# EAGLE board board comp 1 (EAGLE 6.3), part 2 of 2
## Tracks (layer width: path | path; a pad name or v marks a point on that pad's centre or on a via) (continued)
BLINKER_R_FRONT_-  (via drill 0.61) (continued)
  Top 0.254: BLINKER-R1.4 258.95,42.42 | 258.95,42.42 BLINKER-R1.2 | v252.35,28.07 255.65,31.37 255.65,42.42 258.95,42.42
  Bottom 0.254: SV4.15 250.19,12.45 250.19,25.02 252.35,27.18 v252.35,28.07
  pour Top: 255.14,38.99 267.84,38.99 267.84,61.85 255.14,61.85
BRAKE  (via drill 0.61)
  Top 0.254: BRAKE-L1.1 230,41.02 231.39,42.42 237.36,42.42 238.76,41.02 BRAKE-C1.1 238.89,40.89 238.89,35.81 240.41,34.29 243.84,34.29 | 243.84,34.29 243.84,37.08 247.65,40.89 BRAKE-R1.1 | 244.35,27.18 246.13,27.18 247.52,25.78 R9.2 247.52,25.91 247.78,25.91 248.54,26.67 261.87,26.67 262.76,25.78 R16.2 | 244.35,27.18 222.12,27.18 | 222.12,27.18 218.44,27.18 217.04,25.78 R1.2 | v223.39,25.65 224.66,25.65 R3.2 | 222.12,27.18 v222.12,26.92 | 243.84,34.29 244.86,34.29 245.36,33.78 v245.36,29.72 | 244.35,27.18 v244.35,26.8
  Bottom 0.254: v222.12,26.92 v223.39,25.65 | v245.36,29.72 244.35,28.7 v244.35,26.8
BRAKE_C_-  (via drill 0.61)
  Top 0.254: v244.47,33.4 244.47,29.59 244.22,29.34 242.57,29.34 241.17,30.73 BRAKE-C2.2 | v242.95,35.18 241.17,36.96 BRAKE-C2.4 BRAKE-C1.2 BRAKE-C1.4 | SV4.7 240.03,12.45 242.19,12.45 v242.44,12.7
  Bottom 0.254: v242.95,35.18 242.95,34.92 v244.47,33.4 244.35,33.4 242.7,31.75 242.7,26.42 242.82,26.29 242.82,23.11 242.57,22.86 242.57,12.83 v242.44,12.7
  pour Top: 244.98,2.16 244.98,61.85 237.36,61.85 237.36,2.16
BRAKE_L_-  (via drill 0.61)
  Top 0.254: 232.28,39.5 BRAKE-L2.4 232.28,32.26 | 232.28,39.5 BRAKE-L1.2 | 232.28,32.26 BRAKE-L2.2 | v237.11,29.97 237.11,32.26 232.28,32.26 | 232.28,39.5 228.98,39.5 228.98,43.81 232.28,47.12 BRAKE-L1.4
  Bottom 0.254: SV4.9 239.78,12.45 239.78,27.3 v237.11,29.97
  pour Top: 236.09,2.16 236.09,61.85 228.47,61.85 228.47,2.16
BRAKE_R_-  (via drill 0.61)
  Top 0.254: SV4.5 234.7,12.45 234.7,15.49 236.35,15.49 242.44,21.59 v246,21.59 | v249.81,28.07 249.81,30.73 250.06,30.73 BRAKE-R2.2 BRAKE-R2.4 BRAKE-R1.2 BRAKE-R1.4
  Bottom 0.254: v246,21.59 249.81,25.4 v249.81,28.07
  pour Top: 253.87,2.16 253.87,61.85 246.25,61.85 246.25,2.16
BRAKE_REGEN  (via drill 0.61)
  Top 0.254: R2.2 220.85,25.78 221.11,26.04 222.5,26.04 223.01,26.54 227.71,26.54 228.47,25.78 R4.2 228.47,25.91 228.85,26.29 v229.62,26.29 | 231.58,29.15 231.65,29.08 237.49,29.08 238.76,30.35 238.76,30.73 BRAKE-C2.1 238.76,30.23 240.16,28.83 247.65,28.83 | 231.58,29.15 230,30.73 BRAKE-L2.1 | 231.58,29.15 v231.01,28.57 | v245.62,26.29 243.71,24.38 R8.1 | 247.65,28.83 247.65,30.73 BRAKE-R2.1 | 247.65,28.83 v247.65,28.32 248.79,27.18 265.18,27.18 266.57,25.78 R17.2
  Bottom 0.254: v229.62,26.29 231.01,27.69 v231.01,28.57 | v247.65,28.32 v245.62,26.29
CONTACTOR_IN
  Bottom 2.54: CONTACTOR.2 52.45,82.96 K3.S@
CONTACTOR_OUT
  Bottom 2.54: K3.P@ 48.64,87.63 56.26,87.63 56.26,64.14 CONTACTOR.1
CURRENT
  Top 0.254: R84.2 75.31,59.69 SV3.7
D5V+  (via drill 0.61)
  Top 0.254: L5.2 214.12,88.27 214.12,92.08 C53.2 213.64,92.18 C52.2 213.72,95.99 213.72,97.28 213.87,97.28 v218.36,101.78 | v233.45,117.47 233.83,117.09 234.14,117.09 235.03,116.2 R51.2 234.95,116.1 234.95,112.5 C51.2 235.28,112.39 235.28,107.95 U$2.P$27_ | v222.22,112.22 229.11,119.1 v231.88,119.1
  Bottom 0.254: R52.2 233.45,116.31 v233.45,117.47 233.38,117.58 233.38,117.6 v231.88,119.1 | v218.36,101.78 220.96,104.37 220.96,109.65 222.22,110.92 v222.22,112.22
DC+
  Top 0.254: S1.2 194.82,110.13 194.69,110.13 192.56,112.27 192.56,116.2 POWER.1
DGND0  (via drill 0.61)
  Top 0.254: JP11.18 219.15,78.11 220.8,79.76 227.25,79.76 228.91,78.11 JP11.10 229.31,78.11 230.96,79.76 232.99,79.76 | JP11.4 236.53,78.11 234.87,79.76 232.99,79.76 | U$2.P$28_ 235.81,107.95 235.81,108.51 236.45,109.14 C51.1 236.45,112.5 236.45,114.3 235.94,114.81 235.94,119.15 233.12,119.15 231.44,117.47 229.31,117.47 228.22,116.38 227.99,116.38 JP13.6 227.89,116.36 227.89,113.84 JP13.4 227.89,113.72 227.89,111.3 JP13.2 227.74,111.3 223.8,111.3 v222.17,109.68 | C52.1 C53.1 216.74,92.69 221.21,92.69 221.28,92.76 221.39,92.84 | 228.27,94.94 228.27,94.89 228.45,94.89 228.47,94.87 IC10.3 | 228.27,94.94 R53.1 228.27,98.53 228.27,98.7 228.93,99.36 231.19,99.36 231.19,96.06 231.01,95.89 IC10.1 | 228.27,94.94 227.2,94.94 IC10.4 227.1,94.61 223.44,94.61 | 221.39,92.84 222.71,91.52 228.57,91.52 229.39,90.7 229.74,90.7 IC10.7 229.74,88.88 230.63,87.99 231.67,87.99 232.08,88.39 234.77,88.39 234.77,87.2 234.29,86.72 233.66,86.72 233.66,83.08 232.99,82.42 232.99,79.76 | 221.39,92.84 221.39,93.55 222.45,94.61 223.44,94.61 | 223.44,94.61 v223.44,98.65
  Bottom 0.254: v222.17,109.68 222.22,109.63 222.22,99.87 v223.44,98.65
DIR
  Top 0.254: IO.2 160.87,128.78 164.68,124.97 R26.2
DM
  Top 0.254: IC5.7 195.59,9.08 CONN1.D-
DP
  Top 0.254: IC5.8 196.09,12.06 196.34,11.81 CONN1.D+
EECLK  (via drill 0.38)
  Top 0.254: IC5.62 193.97,33.7 v195.2,34.92
  Top 0.305: v190.37,53.21 190.5,53.09 IC7.2 194.06,53.09 194.69,52.45 v200.79,52.45 201.04,52.7 R32.1
  Bottom 0.254: v195.2,34.92 197.49,34.92 200.79,38.23 v200.79,52.45
  Bottom 0.305: JP3.21 189.99,53.59 v190.37,53.21
EECS  (via drill 0.38)
  Top 0.254: IC5.63 194.74,33.2 v195.2,33.66
  Top 0.305: v190.37,51.69 190.5,51.82 IC7.1 193.8,51.82 194.18,51.44 203.07,51.44 v203.45,51.82 203.58,51.94 R34.1
  Bottom 0.254: v195.2,33.66 197.23,33.66 203.33,40.01 203.33,51.69 v203.45,51.82
  Bottom 0.305: JP3.20 189.74,51.05 v190.37,51.69
EEDATA  (via drill 0.38)
  Top 0.254: IC5.61 192.95,34.2 195.2,36.45 v195.71,36.45
  Top 0.305: R31.2 194.5,53.91 194.06,54.36 IC7.3 190.75,54.36 v190.37,54.74
  Bottom 0.254: v195.71,36.45 197.49,36.45 199.52,38.48 199.52,50.16 194.94,54.74 v190.37,54.74
  Bottom 0.305: JP3.22 188.98,56.13 v190.37,54.74
GND  (via drill 0.61)
  Top 0.254: BRAKE-L1.3 234.7,40.89 v236.6,38.99 238.38,37.21 238.38,32.26 242.06,32.26 243.46,30.86 BRAKE-C2.3 | 232.28,24.38 v234.19,24.38 236.09,24.38 R6.1 | 220.85,24.38 217.04,24.38 R1.1 | 228.47,24.38 224.66,24.38 | 224.66,24.38 220.85,24.38 | 220.85,24.38 R2.1 | 224.66,24.38 R3.1 | 228.47,24.38 232.28,24.38 | 232.28,24.38 R5.1 | 228.47,24.38 R4.1 | BLINKER-R1.3 261.24,40.89 v261.24,35.18 261.24,30.86 BLINKER-R2.3 | BRAKE-R1.3 252.35,40.89 v252.35,35.18 252.35,30.86 BRAKE-R2.3 | BLINKER-L1.3 225.68,40.89 v225.68,35.18 225.68,30.86 BLINKER-L2.3 | 258.95,24.38 v257.05,24.38 255.14,24.38 R14.1 | 262.76,24.38 266.57,24.38 R17.1 | 262.76,24.38 258.95,24.38 | 258.95,24.38 R15.1 | 262.76,24.38 R16.1 | v244.86,40.89 243.59,40.89 BRAKE-C1.3 | v235.97,30.73 234.7,30.73 BRAKE-L2.3
  pour Bottom: 267.84,61.85 215.77,61.85 215.77,2.16 267.84,2.16
GND0  (via drill 0.61)
  Top 0.254: v215.14,108.2 R57.2 215.24,109.78 215.62,110.16 218.97,110.16 228.75,119.94 242.72,119.94 245.72,116.94 245.72,113.36 | v211.73,91.47 205.66,85.39 202.95,85.39 201.35,87 R56.2 | 251.71,85.24 259.66,85.24 X3.4 | 251.71,85.24 X3.5 | 251.71,85.24 251.71,78.23 252.68,77.27 254.97,77.27 259.66,72.57 X3.3 | 236.53,102.97 236.78,102.97 U$2.P$11_ | 236.53,102.97 U$2.P$12_ 236.27,102.84 236.27,98.42 C46.1 235.23,98.32 C47.1 235.33,94.54 237.06,92.81 243.56,92.81 243.56,88.67 v244.93,87.3 | 236.8,106.78 236.8,105.74 236.53,105.46 236.53,102.97 | 236.8,106.78 236.8,107.92 U$2.P$30_ | v236.91,106.78 236.8,106.78 | v248.56,112.95 248.56,113.36 245.72,113.36 | 245.72,113.36 240.72,113.36 v238.46,111.1
  Bottom 0.254: v215.14,108.2 213.72,106.78 213.72,95.99 C55.1 C54.1 213.51,92.02 212.95,91.47 v211.73,91.47 | R56.2 200.63,87 200.63,87.12 193.24,94.51 192.38,94.51 192.38,94.54 C57.2 192.28,95.35 192.38,95.45 192.38,97.26 C56.2 195.99,101.04 195.99,102.26 196.65,102.92 196.65,113.26 197.08,113.69 197.08,115.93 POWER.2 | 248.65,112.86 248.84,113.06 253.62,113.06 253.62,113.87 253.67,113.92 253.67,115.09 U$11.4 | 248.65,112.86 248.08,112.29 248.08,112.14 246.89,112.14 C45.1 | C48.1 235.41,109.63 C49.1 235.56,109.63 C50.1 | v236.91,106.78 237.39,107.26 237.39,109.53 C50.1 | v238.46,111.1 238.07,110.72 238.07,109.73 C50.1 | v248.56,112.95 248.65,112.86 | v244.93,87.3 246.96,85.27 X3.5
GND1
  pour Top: 1.65,1.27 99.44,1.27 99.44,50.8 1.65,50.8
GND4
  Top 0.254: U$3.2 216.1,116.36 216.1,112.55 215.14,112.55 R57.1
GND5  (via drill 0.38)
  Top 0.254: ADC_CAP3.2 139.22,46.74 139.79,46.16 | 139.79,46.16 143.76,42.19 ADC3.9 | 7805CAP1.2 108.71,56.26 108.71,52.55 7805CAP2.2 108.69,52.45 106.96,50.72 ADC_CAP1.2 107.06,46.15 119.23,46.15 121.58,43.8 | 126.99,49.14 127.99,50.14 129.01,50.14 | 126.99,49.14 124.08,46.23 ADC_CAP2.2 123.95,46.18 121.58,43.8 | 129.01,50.14 129.79,50.93 6103CAP2.2 129.87,51.03 130.18,51.33 130.18,54.63 3V.3 129.82,55.17 6103CAP1.2 129.92,58.62 131.29,59.99 142.26,59.99 317CAP2.2 142.37,60.07 145.54,60.07 146.43,59.18 317CAP1.2 146.48,59.05 149.22,56.31 R22.2 149.33,54.86 160.07,54.86 162.13,52.81 162.13,52.25 U$1.4 162.18,46.18 160.11,44.11 | 121.58,43.8 120.98,43.2 117.55,43.2 115.95,41.6 115.82,41.6 ADC1.9 | v130.71,42.52 129.79,41.6 ADC2.9 | 130.71,46.86 130.71,48.41 129.08,50.04 129.01,50.14 | 130.71,46.86 v130.71,46.18 | 130.71,46.86 v135.18,46.86 | v139.65,46.02 139.79,46.16 | 126.99,49.14 121.64,54.48 5V.3 | ADC_CAP4.2 154.15,46.23 157.73,42.65 ADC4.9 157.84,41.83 160.11,44.11 | 169.48,34.73 SV2.2 SV2.3 | 169.48,34.73 166.32,31.57 166.32,24.89 R23.2 166.24,24.79 166.24,15.34 160.27,9.37 SV1.33 | 169.48,34.73 160.11,44.11
  Bottom 0.254: v130.71,46.18 v130.71,42.52 | v139.65,46.02 136.02,46.02 v135.18,46.86
  pour Bottom: 103.12,40.77 103.12,70.61 176.78,70.61 176.78,1.4 165.99,1.4 165.99,40.77
  pour Top: 103.12,40.77 103.12,70.61 176.78,70.61 176.78,1.4 165.99,1.4 165.99,40.77
GND6
  Top 0.254: 169.13,118.62 169.13,119.89 164.05,119.89 162.78,118.62 T1.2 | 169.13,118.62 167.86,117.35 167.86,95.76 165.32,93.22 POWER1.1 | 169.13,118.62 T2.2
  Bottom 2.794: POWER1.1 156.43,92.58 156.43,95.76 137.05,95.76 K2.P2
GND7  (via drill 0.38)
  Top 0.254: IC5.15 199.59,32.64 v199.64,32.64 198.75,32.64 198.59,32.48 IC5.13 | IC5.11 197.59,32.02 197.49,32.13 194.94,32.13 194.59,31.78 IC5.5 | IC5.1 192.59,31.81 192.66,31.88 194.18,31.88 | IC5.47 193.09,43.13 192.91,43.31 v192.28,43.31 | IC5.51 196,39.2 196.22,38.99 196.22,38.1 v196.09,37.97 | IC5.35 199.09,40.68 199.26,40.51 200.28,40.51 200.91,41.15 v202.06,41.15 | IC5.25 208.66,36.7 210.19,35.18 | 197.1,30.86 197.1,31.88 | 198.59,30.9 198.59,29.7 199.35,28.94
  other vias: 204.72,15.88 207.77,15.88 209.04,11.56 197.99,12.57 198.88,8.51 207.77,30.1 203.96,19.68 190.75,29.34 188.72,23.5 205.23,22.73 190.25,17.91 202.18,43.81 202.18,49.66 191.9,6.1 189.48,10.41 198.75,22.99 199.9,28.07 192.02,11.18 194.18,4.32 197.99,4.06 196.22,1.78 201.55,12.19 188.85,6.1 202.31,57.15 207.65,57.15 206.63,41.91 208.41,42.16 202.31,31.5 185.29,47.24 182.75,54.86 185.04,55.12
  pour Bottom (isolate 0.305): 213.49,0.89 213.49,58.04 179.2,58.04 179.2,0.89
  pour Top (isolate 0.305): 213.49,0.89 213.49,58.04 179.2,58.04 179.2,0.89
GND8  (via drill 0.6)
  other vias: 65.15,113.03 43.56,100.33 66.42,119.38 62.61,77.47
  pour Top: 1.65,54.61 99.44,54.61 99.44,139.7 1.65,139.7
  pour Bottom: 1.65,54.61 99.44,54.61 99.44,139.7 1.65,139.7
IN1  (via drill 0.38)
  Top 0.254: 110.74,20.7 110.74,17.27 SV1.1 | 110.74,20.7 LMC6484_1.3 | v119.63,22.17 120.37,22.91 124.08,22.91 U$6.1 | 110.74,20.7 v118.16,20.7
  Bottom 0.254: v118.16,20.7 v119.63,22.17
IN2
  Top 0.254: LMC6484_1.5 113.28,22.58 114.43,21.44 119.63,21.44 | 119.63,21.44 124.46,21.44 125.35,22.33 U$6.2 | 119.63,21.44 SV1.2
IN3  (via drill 0.38)
  Top 0.254: SV1.3 123.27,9.47 123.27,11.02 126.62,14.38 U$6.3 126.57,23.04 126.57,23.6 125.53,24.64 v124.38,24.64 | LMC6484_1.10 113.28,27.76 114.55,26.49 v122.53,26.49
  Bottom 0.254: v124.38,24.64 v122.53,26.49
IN4  (via drill 0.38)
  Top 0.254: U$6.4 127.89,16.69 v127.36,16.15 | v124.51,13.31 124.51,13.26 SV1.4 | LMC6484_1.12 110.74,27.08 v112.93,24.89
  Bottom 0.254: v127.36,16.15 v124.51,13.31 v112.93,24.89
IN5  (via drill 0.38)
  Top 0.254: U$6.5 129.16,16.41 v128.35,15.6 | ADC1.5 112.01,35.79 v119.84,27.96
  Bottom 0.254: SV1.5 125.81,9.47 127.36,9.47 128.35,10.46 v128.35,15.6 128.27,15.7 128.27,21.79 122.1,27.96 v119.84,27.96
IN6  (via drill 0.38)
  Top 0.254: SV1.6 130.43,16.64 U$6.6 130.38,23.04 130.38,23.6 v129.34,24.64 | ADC1.6 113.28,35.79 v120.12,28.96
  Bottom 0.254: v120.12,28.96 125.02,28.96 v129.34,24.64
IN7  (via drill 0.38)
  Top 0.254: SV1.7 128.35,9.47 128.35,11.02 131.93,14.61 131.93,21.01 131.7,21.23 U$6.7 131.65,23.04 131.65,23.6 v130.43,24.82 | ADC1.7 114.55,35.79 v120.4,29.95
  Bottom 0.254: v120.4,29.95 125.3,29.95 v130.43,24.82
IN8  (via drill 0.38)
  Top 0.254: ADC1.8 115.82,35.56 v116.61,34.77 | v132.97,25.91 U$6.9 | v131.19,20.7 131.19,14.86 SV1.8
  Bottom 0.254: v116.61,34.77 116.61,24.77 116.18,24.33 114.53,24.33 113.23,25.63 112.62,25.63 112.19,25.2 112.19,24.59 124.77,12.01 126.16,12.01 SV1.8 | v132.97,25.91 132.97,22.48 v131.19,20.7
IN9  (via drill 0.38)
  Top 0.254: v131.7,30.61 U$6.10 | v121.54,38 121.54,37.03 ADC2.1
  Bottom 0.254: v131.7,30.61 131.7,30.89 128.08,34.51 | 128.08,34.51 124.59,38 v121.54,38 | SV1.9 130.78,8.38 132.23,9.83 135.33,9.83 136.32,10.82 136.32,15.14 142.09,20.9 142.09,23.6 131.09,34.59 128.17,34.59 128.08,34.51
IN10  (via drill 0.38)
  Top 0.254: v130.43,26.42 U$6.11 | v122.17,34.65 ADC2.2
  Bottom 0.254: SV1.10 129.79,23.11 131.17,24.49 131.17,25.12 130.43,25.86 v130.43,26.42 130.33,26.49 v122.17,34.65
IN11
  Top 0.254: ADC2.3 123.44,37.01 124.92,38.48 130.53,38.48 131.19,37.82 131.19,32.05 | 131.19,32.05 131.19,31.14 129.16,29.11 U$6.12 | SV1.11 132.33,9.37 133.66,10.69 133.66,25.65 133.71,25.7 133.71,29.64 131.29,32.05 131.19,32.05
IN12  (via drill 0.38)
  Top 0.254: 127.89,29.84 127.89,30.91 130.53,33.55 130.53,37.54 130.25,37.82 125.53,37.82 124.71,37.01 ADC2.4 | 127.89,29.84 U$6.13 | v128.04,29.84 127.89,29.84
  Bottom 0.254: SV1.12 132.33,18.52 130.45,20.4 130.45,22.84 131.83,24.21 131.83,26.06 v128.04,29.84
IN13  (via drill 0.38)
  Top 0.254: ADC2.5 125.98,34.52 126.62,33.88 U$6.14 126.57,28.02 126.57,27.46 125.81,26.7 123.62,26.7 123.09,27.23 v121.08,27.23 | SV1.13 133.88,8.38 132.79,7.29 121.72,7.29 121.08,7.92 v121.08,20.7
  Bottom 0.254: v121.08,27.23 v121.08,20.7
IN14  (via drill 0.38)
  Top 0.254: v125.35,33.15 U$6.15 | v126.87,34.67 126.87,35.99 127.25,36.37 ADC2.6
  Bottom 0.254: v126.87,34.67 126.21,34.01 | 126.21,34.01 v125.35,33.15 | SV1.14 134.87,22.12 135.13,22.38 135.13,25.09 126.21,34.01
IN15  (via drill 0.38)
  Top 0.254: SV1.15 136.32,9.47 136.32,11.38 138.05,13.11 U$7.1 138,23.04 137.13,23.9 v137.13,24.13 | v128.52,32.74 ADC2.7
  Bottom 0.254: v137.13,24.13 v128.52,32.74
IN16  (via drill 0.38)
  Top 0.254: SV1.16 139.32,12.83 U$7.2 139.27,23.04 138.96,23.34 v138.96,24.64 | v129.79,33.86 ADC2.8
  Bottom 0.254: v129.79,33.86 129.79,33.81 v138.96,24.64
IN17  (via drill 0.38)
  Top 0.254: SV1.17 138.86,9.47 138.86,11.38 140.59,13.11 U$7.3 140.54,23.04 140.03,23.55 v140.03,24.61 | v134.87,29.77 ADC3.1
  Bottom 0.254: v140.03,24.61 v134.87,29.77
IN18  (via drill 0.38)
  Top 0.254: 141.86,21.21 141.86,12.83 SV1.18 | 141.86,21.21 U$7.4 | v136.14,26.42 ADC3.2 | 141.86,21.21 v141.35,21.21
  Bottom 0.254: v141.35,21.21 v136.14,26.42
IN19  (via drill 0.38)
  Top 0.254: SV1.19 141.4,9.47 141.4,11.38 143.13,13.11 U$7.5 143.08,23.04 142.54,23.57 v142.54,24.61 | v137.41,29.74 ADC3.3
  Bottom 0.254: v142.54,24.61 v137.41,29.74
IN20  (via drill 0.38)
  Top 0.254: SV1.20 144.4,12.83 U$7.6 144.35,23.04 144.35,23.6 143.56,24.38 v143.56,24.64 | v138.68,32.05 ADC3.4
  Bottom 0.254: v138.68,32.05 139.37,31.37 139.37,30.4 139.12,30.15 139.12,29.08 v143.56,24.64
IN21  (via drill 0.38)
  Top 0.254: SV1.21 143.94,9.47 143.94,11.38 145.67,13.11 U$7.7 145.62,23.04 145.62,23.62 v144.6,24.64 | ADC3.5 139.95,31.7 v140.08,31.57
  Bottom 0.254: v140.08,31.57 140.08,29.16 v144.6,24.64
IN22  (via drill 0.38)
  Top 0.254: U$7.9 146.94,29.79 v145.8,30.94 | v143.66,33.07 143.66,33.17 141.22,35.61 ADC3.6 | SV1.22 145.03,11.53 146.41,12.9 v146.41,17.68
  Bottom 0.254: v143.66,33.07 144.21,32.52 | 144.21,32.52 v145.8,30.94 | v146.41,17.68 146.41,24.79 141.76,29.44 141.76,30.07 144.21,32.52
IN23  (via drill 0.38)
  Top 0.254: U$7.10 145.67,30.02 145.06,30.63 145.06,31.24 145.49,31.67 146.1,31.67 147.6,30.18 147.6,29.11 148.03,28.68 148.64,28.68 | 148.64,28.68 149.07,29.11 149.07,31.37 144.42,36.02 144.42,37.62 144.22,37.82 143.31,37.82 142.49,37.01 ADC3.7 | v148.67,28.42 148.67,28.57 148.64,28.68
  Bottom 0.254: SV1.23 147.57,9.37 148.67,10.46 v148.67,28.42
IN24  (via drill 0.38)
  Top 0.254: 144.4,32.33 144.4,35.1 143.76,35.74 ADC3.8 | 144.4,32.33 U$7.11 | v148.34,29.41 148.34,30.38 146.38,32.33 144.4,32.33
  Bottom 0.254: SV1.24 147.57,28.65 v148.34,29.41
IN25  (via drill 0.38)
  Top 0.254: U$7.12 143.13,29.31 v143.66,29.84 | v148.9,34.67 148.9,36.32 148.84,36.37 ADC4.1
  Bottom 0.254: v143.66,29.84 145.75,29.84 148.9,32.99 148.9,34.01 | v148.9,34.67 148.9,34.01 | SV1.25 150.11,9.37 151.21,10.46 151.21,33.22 150.42,34.01 148.9,34.01
IN26  (via drill 0.38)
  Top 0.254: U$7.13 141.86,29.11 v142.49,29.74 | ADC4.2 v150.11,33.27
  Bottom 0.254: v142.49,29.74 142.72,29.74 143.36,29.11 145.95,29.11 147.81,30.98 | v150.11,33.27 147.81,30.98 | SV1.26 150.11,28.68 147.81,30.98
IN27  (via drill 0.38)
  Top 0.254: U$7.14 140.59,31.04 v142.67,33.12 | v150.85,34.67 150.85,35.84 151.38,36.37 ADC4.3 151.28,36.45 151.28,38.3 151.71,38.73 v154.31,38.73
  Bottom 0.254: v142.67,33.12 144.96,35.41 150.11,35.41 v150.85,34.67 | SV1.27 153.65,8.38 154.74,7.29 160.73,7.29 161.37,7.92 161.37,31.67 v154.31,38.73
IN28  (via drill 0.38)
  Top 0.254: U$7.15 139.32,30.38 v138.63,31.06 | v152.76,34.67 152.76,36.27 152.65,36.37 ADC4.4
  Bottom 0.254: v138.63,31.06 137.95,31.75 137.95,32.36 143.26,37.67 150.65,37.67 151.71,38.73 152.32,38.73 152.76,38.3 v152.76,34.67 152.76,24.51 152.65,24.41 SV1.28
IN29  (via drill 0.38)
  Top 0.254: U$8.1 152.02,14.15 v154.1,12.06 | v153.92,34.29 ADC4.5
  Bottom 0.254: SV1.29 154.1,9.47 v154.1,12.06 154.03,12.17 153.92,12.27 v153.92,34.29
IN30  (via drill 0.38)
  Top 0.254: SV1.30 155.19,12.01 153.29,13.92 U$8.2 153.24,23.04 153.24,23.6 v152.02,24.82 | ADC4.6 155.19,37.01 154.2,38 v152.02,38
  Bottom 0.254: v152.02,24.82 v152.02,38
IN31  (via drill 0.38)
  Top 0.254: ADC4.7 156.46,35.79 153.92,33.25 153.92,26.87 154.56,26.24 U$8.3 154.61,22.81 154.61,22.28 v156.29,20.6
  Bottom 0.254: SV1.31 157.73,9.37 156.29,10.82 v156.29,20.6
IN32  (via drill 0.38)
  Top 0.254: U$8.5 155.83,33.88 157.73,35.79 ADC4.8 157.78,36.5 158.37,37.08 v158.37,38 | v158.37,43.41 U$1.1
  Bottom 0.254: v158.37,38 v158.37,43.41
MOTOR+
  Top 2.794: OUTPUT.2 142.46,133.86 D2.C
MOTOR+_PRE
  Bottom 2.794: K1.O2 132.06,83.19 132.06,86.98 142.05,86.98 K1.S1 152.62,90.68 152.62,88.14 171.67,88.14 171.67,104.65 157.7,104.65 D2.A
MOTOR-
  Top 2.794: OUTPUT.1 118.33,133.86 D1.C
MOTOR-_PRE
  Top 2.794: D1.A 132.07,117.35 K1.O1
  Bottom 2.794: K1.O1 128.49,90.68 128.49,79.25 142.05,79.25 K1.S2
N$1
  Top 0.254: SV4.2 231.01,17.53 236.98,23.5 236.98,24.13 239.27,26.42 240.54,26.42 241.05,25.91 243.59,25.91 243.71,25.78 R8.2
N$2  (via drill 0.61)
  Top 0.254: v232.16,15.11 232.16,17.91 239.9,25.65 R7.2
  Bottom 0.254: v232.16,15.11 233.55,13.72 SV4.4
N$3  (via drill 0.61)
  Top 0.254: v241.94,23.5 246.76,23.5 247.52,24.26 R9.1 | v240.66,22.23 233.17,14.73 233.04,14.73 232.16,13.84 232.16,11.05 SV4.1
  Bottom 0.254: v240.66,22.23 v241.94,23.5
N$4  (via drill 0.61)
  Top 0.254: v249.05,23.37 250.44,23.37 251.33,24.26 R10.1 | v247.27,21.59 240.54,14.86 v236.98,14.86
  Bottom 0.254: v247.27,21.59 v249.05,23.37 | v236.98,14.86 235.33,14.86 235.33,14.48 234.7,13.84 234.7,12.32 233.55,11.18 SV4.3
N$5
  Top 0.254: R11.2 4.19,29.97 | 4.19,29.97 R12.1 | 4.19,29.97 6.86,29.97 IC2.1
N$6
  Top 0.254: R13.2 70.23,38.86 | 70.23,38.86 R18.1 | 70.23,38.86 72.9,38.86 IC1.1
N$7
  Top 0.254: R20.1 96.9,30.99 | 96.9,30.99 R19.2 | 96.9,30.99 94.23,30.99 IC3.1
N$8
  Top 0.254: R21.2 138.43,53.39 IC4.1 141.55,50.44 144.15,53.03 149.22,53.03 R22.1
N$9
  Top 2.794: K1.P2 137.12,83.19 137.12,79.01 146.27,79.01 146.27,107.19 K2.S1
N$10
  Top 2.794: K1.P1 137.38,90.68 137.38,95.76 142.05,95.76 K2.S2
N$11
  Top 0.254: R24.1 151.35,112.27 150.84,112.78 133.82,112.78 133.82,89.53 127.47,83.19 K1.1
N$12  (via drill 0.61)
  Top 0.254: v168.75,102.49 168.75,111.38 169.63,112.27 R25.1
  Bottom 0.254: v168.75,102.49 168.36,102.11 119.47,102.11 K2.1
N$13
  Top 0.254: K1.2 127.22,100.84 127.22,136.4 143.73,136.4 164.05,116.08 T1.1
N$14  (via drill 0.61)
  Top 0.254: v169.13,116.08 170.4,116.08 T2.1
  Bottom 0.254: v169.13,116.08 165.32,119.89 129.76,119.89 K2.2
N$15
  Top 0.254: T2.3 171.28,118.36 169.76,119.89 R27.1
N$16  (via drill 0.61)
  Top 0.254: T1.3 167.47,118.36 v167.47,119 | v167.47,120.9 163.41,124.97 R26.1
  Bottom 0.254: v167.47,120.9 v167.47,119
N$17
  Top 0.254: IC5.6 195.09,17.29 193.93,16.13 R29.2
N$18
  Top 0.254: IC5.2 193.09,28.88 191.64,27.43 191.64,26.29 X1.1
  Top 0.305: C11.1 188.34,26.8 188.59,26.54 191.39,26.54 191.64,26.29
N$19
  Top 0.254: IC5.3 193.59,21.25 193.04,20.7 X1.2
  Top 0.305: C12.1 188.41,19.75 188.59,19.94 188.59,20.19 191.13,20.19 X1.2
N$20
  Top 0.406: PWR.C R28.2
N$21
  Top 0.305: R35.2 RX.C
N$22
  Top 0.305: R36.2 TX.C
N$23
  Top 0.254: U$2.P$1_ 238.53,107.21 243,111.68 250.39,111.68 C41.1 250.8,112.06 252.04,112.06 252.37,112.39 R40.2
N$24
  Top 0.254: U$2.P$2_ 238.53,106.7 247.17,106.7 250.7,110.24 C41.2 250.8,110.16 252.07,110.16 252.37,109.86 R41.2
N$25
  Top 0.254: U$2.P$3_ 238.53,106.2 250.16,106.2 250.7,105.66 C42.1 250.8,105.59 251.23,105.16 253.19,105.16 254.08,106.05 R42.2
N$26  (via drill 0.61)
  Top 0.254: v237.36,105.11 237.95,105.69 238.51,105.69 U$2.P$4_ | v238.68,102.84 238.96,102.56 249.38,102.56 250.7,103.89 C42.2 250.67,103.68 251.74,102.62 253.19,102.62 254.08,103.5 R43.2
  Bottom 0.254: v237.36,105.11 238.68,103.78 v238.68,102.84
N$27  (via drill 0.61)
  Top 0.254: v244.98,105.21 238.53,105.21 U$2.P$5_ | v245.09,100.89 245.39,100.58 250.7,100.58 C43.1 250.8,100.66 252.07,100.66 252.37,100.97 R44.2
  Bottom 0.254: v244.98,105.21 245.09,105.11 v245.09,100.89
N$28  (via drill 0.61)
  Top 0.254: v249.4,104.24 244.75,104.24 244.3,104.7 238.53,104.7 U$2.P$6_ | v249.5,99.75 250.42,98.83 250.7,98.83 C43.2 250.8,98.75 252.04,98.75 252.37,98.42 R45.2
  Bottom 0.254: v249.4,104.24 249.66,103.99 249.66,99.9 v249.5,99.75
N$29  (via drill 0.61)
  Top 0.254: v248.51,103.4 244.93,103.4 244.09,104.24 242.29,104.24 242.26,104.22 238.53,104.22 U$2.P$7_ | v248.82,101.73 248.94,101.85 253.03,101.85 253.24,101.65 253.24,95.89 R46.2 252.27,95.83 251.03,95.83 250.7,95.5 C44.1
  Bottom 0.254: v248.51,103.4 248.82,103.1 v248.82,101.73
N$30  (via drill 0.61)
  Top 0.254: v242.65,103.4 242.37,103.68 238.53,103.68 U$2.P$8_ | v243.56,100.89 250.7,93.75 C44.2 250.8,93.67 252.04,93.67 252.37,93.34 R47.2
  Bottom 0.254: v242.65,103.4 243.56,102.49 v243.56,100.89
N$31  (via drill 0.61)
  Top 0.254: 251.66,116.94 251.66,118.75 JP7.1 | 251.66,116.94 251.66,114.81 254.08,112.39 R40.1 | 251.66,116.94 v249.81,116.94
  Bottom 0.254: R48.2 249.83,118.75 249.81,118.72 v249.81,116.94 249.81,116.36 249.86,116.31 249.86,115.11 U$11.1
N$32
  Bottom 0.254: R48.1 251.54,118.75 251.44,118.64 251.44,117.2 251.08,116.84 251.08,116.36 251.13,116.31 251.13,115.11 U$11.2
N$33  (via drill 0.61)
  Top 0.254: v252.5,116.94 252.55,116.99 260.38,116.99 JP7.3
  Bottom 0.254: v252.5,116.94 252.5,115.19 U$11.3
N$34  (via drill 0.61)
  Top 0.254: JP8.1 257.05,112.8 254.1,109.86 R41.1 254.03,109.96 v252.86,111.12
  Bottom 0.254: R49.2 251.1,104.78 251.08,104.8 251.08,106.66 251.16,106.73 251.16,107.92 U$11.7 251.18,108.05 251.23,108.1 251.23,109.5 v252.86,111.12
N$35
  Bottom 0.254: R49.1 252.81,104.78 252.71,104.88 252.71,106.17 252.5,106.38 252.5,106.66 252.43,106.73 252.43,107.92 U$11.6
N$36  (via drill 0.61)
  Top 0.254: v254.71,107.92 255.09,107.54 262,107.54 262.61,108.15 262.61,114.94 JP8.3
  Bottom 0.254: v254.71,107.92 253.69,107.92 U$11.5
N$37
  Top 0.254: JP14.2 259.97,106.93 253.29,106.93 R42.1
N$38
  Top 0.254: JP14.1 259.97,104.39 253.29,104.39 R43.1
N$39
  Top 0.254: JP15.4 R44.1
N$40
  Top 0.254: JP15.3 R45.1
N$41
  Top 0.254: JP15.2 R46.1
N$42
  Top 0.254: JP15.1 R47.1
N$43  (via drill 0.61)
  Top 0.254: 237.79,100.89 237.79,98.42 C46.2 | 237.79,100.89 U$2.P$9_ | 237.79,100.89 v240.41,100.89
  Bottom 0.254: JP9.2 239.27,114.94 239.27,114.45 240.41,113.31 v240.41,100.89
N$44  (via drill 0.61)
  Top 0.254: v244.86,112.52 242.37,112.52 237.79,107.95 U$2.P$32_ | v244.88,116.59 242.95,118.52 239.04,118.52 JP9.1
  Bottom 0.254: v244.86,112.52 244.88,112.55 v244.88,116.59
N$45
  Top 0.305: IC7.4 196.15,55.63 R31.1 196.66,55.56 197.23,54.99 197.23,54.23 197.49,53.98 198.25,53.98 R33.1
N$46
  Top 0.254: JP10.2 240.06,117.47 240.06,114.07 237.31,111.33 237.31,107.95 U$2.P$31_
N$47  (via drill 0.61)
  Top 0.254: 237.13,96.62 237.13,94.61 C47.2 | 237.13,96.62 237.13,100 237.29,100.15 U$2.P$10_ | v241.81,100.89 239.32,98.4 239.32,96.62 237.13,96.62
  Bottom 0.254: JP10.1 242.59,114.15 242.59,113.77 243.81,112.55 243.81,112.32 244.88,111.25 244.88,106.83 241.81,103.76 v241.81,100.89
N$48
  Top 0.254: IC5.4 194.09,19.09 191.13,16.13 C16.1
  Top 0.406: C16.1 191.46,15.05 191.13,15.37 189,15.37 | 188.7,15.37 C14.+ 189,15.37 | L2.1 186.91,14.95 187.32,15.37 188.7,15.37 | 189,15.37 188.7,15.37
N$49
  Top 0.254: IC5.9 196.59,23.37 197.87,22.1 C15.1 197.93,20.38 198.25,20.7
  Top 0.305: 198.25,20.7 199.79,20.7 C13.+ 200.05,20.93 200.28,20.7 201.76,20.7 L1.1
N$50  (via drill 0.61)
  Top 0.254: v234.72,105.11 234.11,105.72 U$2.P$21_ | v242.72,91.24 242.72,75.64 240.16,75.64 240.08,75.56 JP11.1
  Bottom 0.254: v234.72,105.11 244.88,94.94 244.88,93.12 244.37,92.61 242.54,92.61 242.54,91.42 v242.72,91.24
N$51  (via drill 0.61)
  Top 0.254: v231.93,106.86 232.56,106.22 233.55,106.22 U$2.P$22_
  Bottom 0.254: v231.93,106.86 231.65,106.58 R50.1
N$52
  Top 0.254: JP11.5 234.26,75.64 235.84,75.64 235.91,75.56 JP11.3
  Bottom 0.254: JP11.3 236.73,75.46 237.74,74.45 237.74,73.91 239.95,73.91 242.34,76.3 242.34,90.42 241.88,90.88 241.88,91.9 231.83,101.96 231.83,103.73 231.65,103.91 R50.2
N$53  (via drill 0.61)
  Top 0.254: JP11.9 229.18,75.64 230.76,75.64 230.84,75.56 JP11.7 | JP12.1 229.87,107.31 231.95,105.23 233.55,105.23 U$2.P$20_ | v232.03,89.23 232.03,99.9 v226.64,99.9
  Bottom 0.254: JP11.7 233.15,77.06 233.15,78.54 233.3,78.69 233.3,78.79 231.6,80.49 231.6,88.8 v232.03,89.23 | v226.64,99.9 225.43,101.12 225.43,105.49 227.25,107.31 JP12.1
N$54  (via drill 0.61)
  Top 0.254: v230.35,103.68 230.86,104.19 233.55,104.19 U$2.P$18_
  Bottom 0.254: v230.35,103.68 230.15,103.48 230.15,102.74 230.91,101.98 230.91,95.66 228.32,93.07 228.32,79.65 227.46,78.79 227.46,78.69 227.61,78.54 227.61,77.67 227.46,77.52 227.46,77.32 227.58,77.19 227.58,76.78 226.57,75.77 JP11.11
N$55  (via drill 0.61)
  Top 0.254: v231.9,113.56 231.9,113.03 233.68,111.25 234.29,111.25 234.29,107.95 U$2.P$25_ | v227.91,109.86 227.31,109.25 224.51,109.25 222.02,106.76 222.02,102.03 v221.39,102.03
  Bottom 0.254: v231.9,113.56 231.47,113.56 231.47,113.41 230.4,112.34 229.82,112.34 229.82,112.19 228.93,111.3 228.93,110.87 v227.91,109.86 | v221.39,102.03 221.77,101.65 221.77,99.67 222.22,99.21 222.22,84.33 224.89,81.66 224.89,78.72 225.07,78.54 225.07,77.67 224.92,77.52 224.92,77.32 225.04,77.19 225.04,76.78 224.03,75.77 JP11.13
N$56  (via drill 0.61)
  Top 0.254: v234.72,106.5 234.31,106.5 234.14,106.68 233.6,106.68 U$2.P$23_ | v234.26,100.71 234.26,100.15 233.66,99.54 v233.66,89.23 | v232.44,87.55 227.33,82.45 225.81,82.45 v223.95,80.59
  Bottom 0.254: v234.72,106.5 233.88,105.66 233.88,103.58 234.26,103.2 v234.26,100.71 | v233.66,89.23 232.44,88.01 v232.44,87.55 | v223.95,80.59 222.99,79.63 222.99,77.67 223.14,77.52 223.14,77.42 221.49,75.77 JP11.15
N$57  (via drill 0.61)
  Top 0.254: v229.82,106.17 231.27,104.72 233.55,104.72 U$2.P$19_
  Bottom 0.254: v229.82,106.17 228.42,104.78 JP12.2
N$58  (via drill 0.61)
  Top 0.254: v227.48,86.69 223.24,82.45 221.82,82.45 217.91,78.54 217.91,76.38 217.93,76.38 218.75,75.56 JP11.17
  Bottom 0.254: JP12.3 227.48,101.88 v227.48,86.69
N$59  (via drill 0.61)
  Top 0.254: v229.13,109.88 228.04,108.79 224.71,108.79 224.71,104.5 225.48,103.73 229.11,103.73 230.84,102.01 234.29,102.01 U$2.P$16_
  Bottom 0.254: v229.13,109.88 230.4,111.15 230.4,111.28 JP13.1
N$60  (via drill 0.61)
  Top 0.254: v233.43,102.84 233.55,102.84 233.55,103.68 U$2.P$17_ | v233.4,108.23 233.4,110.87 230.45,113.82 230.43,113.82 JP13.3 230.78,113.67 233.32,116.2 R51.1
  Bottom 0.254: v233.43,102.84 233.4,102.87 v233.4,108.23
N$61  (via drill 0.61)
  Top 0.254: U$2.P$24_ 233.55,107.21 233.38,107.39 232.82,107.39 229.36,110.85 229.36,116.36 230.4,116.36 JP13.5 230.53,116.41 231.04,116.41 232.94,118.31 234.11,118.31 v234.95,117.47
  Bottom 0.254: v234.95,117.47 234.95,116.28 235.03,116.2 R52.1
N$62
  Top 0.254: JP11.20 216.46,78.11 216.46,78.87 221.72,84.12 221.87,84.12 227.2,89.46 IC10.5
N$63  (via drill 0.61)
  Top 0.254: v222.07,83.29 226.31,87.53 227.84,87.53 227.84,88.82 228.47,89.46 IC10.6
  Bottom 0.254: v222.07,83.29 222.02,83.24 222.02,80.06 221.41,79.45 221.41,78.99 221.49,78.92 JP11.16
N$64  (via drill 0.61)
  Top 0.254: C57.1 194.72,87.1 196.52,87.1 196.62,87 R55.1 197.46,87.07 198.98,88.59 203.2,88.59 204.8,87 R54.1 | v215.14,89.28 216.15,88.27 L5.1
  Bottom 0.254: v215.14,89.28 215.14,89.26 L6.2 214.02,88.21 206.81,88.21 | 206.81,88.21 205.97,88.21 205.97,88.01 204.98,87.02 R54.1 | IC15.2 206.4,102.08 206.4,100.13 206.81,99.72 206.81,88.21
N$65
  Top 0.254: R55.2 197.46,97.26 200.33,97.26 200.43,97.16 R56.1
  Bottom 0.254: IC15.1 203.56,102.08 203.56,100.13 201.17,97.74 R56.1
N$66
  Top 0.254: C56.1 191.01,101.5 191.26,101.5 198.35,108.58 S1.1
  Bottom 0.254: IC15.3 208.08,102.95 208.08,103.76 203.35,108.48 198.63,108.48 S1.1
N$67
  pour Bottom: 221.49,121.28 221.49,83.19 188.47,83.19 188.47,121.28
N$68
  pour Top: 221.49,121.28 221.49,83.19 188.47,83.19 188.47,121.28
N$69
  pour Bottom: 263.4,92.08 263.4,67.94 243.08,67.94 243.08,92.08 245.62,92.08 245.62,120.02 255.78,120.02 255.78,92.08
  pour Bottom: 255.78,92.08 259.59,92.08 259.59,113.67 255.78,113.67
N$70
  pour Bottom: 244.35,120.02 244.35,93.34 241.81,93.34 241.81,83.19 222.76,83.19 222.76,120.02
N$71
  pour Bottom: 241.81,81.92 241.81,67.94 189.74,67.94 189.74,81.92
N$72
  pour Top: 241.81,90.81 241.81,67.94 189.74,67.94 189.74,81.92 234.19,81.92 234.19,90.81
N$73
  pour Top: 240.54,109.86 240.54,100.97 231.65,100.97 231.65,109.86
N$74
  Top 0.508: U$5.P$1 NEWBATT.P$2
  Bottom 0.508: OLDBATT.P$2 U$5.P$1
N$75
  Top 0.508: U$9.P$1 NEWBATT.P$1
  Bottom 0.508: OLDBATT.P$1 U$9.P$1
N$76
  pour Top: 186.56,124.71 186.56,138.94 196.22,138.94 196.22,124.71
N$77
  pour Bottom: 186.56,124.71 186.56,138.94 196.22,138.94 196.22,124.71
N$78
  Top 0.508: U$10.P$1 NEWBATT1.P$2
  Bottom 0.508: OLDBATT1.P$2 U$10.P$1
N$79
  Top 0.508: U$12.P$1 NEWBATT1.P$1
  Bottom 0.508: OLDBATT1.P$1 U$12.P$1
N$80
  pour Top: 198.63,124.71 198.63,138.94 208.28,138.94 208.28,124.71
N$81
  pour Bottom: 198.63,124.71 198.63,138.94 208.28,138.94 208.28,124.71
N$82
  Top 0.508: U$13.P$1 NEWBATT2.P$2
  Bottom 0.508: OLDBATT2.P$2 U$13.P$1
N$83
  Top 0.508: U$14.P$1 NEWBATT2.P$1
  Bottom 0.508: OLDBATT2.P$1 U$14.P$1
N$84
  pour Top: 210.57,124.71 210.57,138.94 220.22,138.94 220.22,124.71
N$85
  pour Bottom: 210.57,124.71 210.57,138.94 220.22,138.94 220.22,124.71
N$86
  Top 0.508: U$15.P$1 NEWBATT3.P$2
  Bottom 0.508: OLDBATT3.P$2 U$15.P$1
N$87
  Top 0.508: U$16.P$1 NEWBATT3.P$1
  Bottom 0.508: OLDBATT3.P$1 U$16.P$1
N$88
  pour Top: 222.38,124.71 222.38,138.94 232.03,138.94 232.03,124.71
N$89
  pour Bottom: 222.38,124.71 222.38,138.94 232.03,138.94 232.03,124.71
N$90
  Top 0.508: U$17.P$1 NEWBATT4.P$2
  Bottom 0.508: OLDBATT4.P$2 U$17.P$1
N$91
  Top 0.508: U$18.P$1 NEWBATT4.P$1
  Bottom 0.508: OLDBATT4.P$1 U$18.P$1
N$92
  pour Top: 234.19,124.71 234.19,138.94 243.84,138.94 243.84,124.71
N$93
  pour Bottom: 234.19,124.71 234.19,138.94 243.84,138.94 243.84,124.71
N$94
  Top 0.508: U$19.P$1 NEWBATT5.P$2
  Bottom 0.508: OLDBATT5.P$2 U$19.P$1
N$95
  Top 0.508: U$20.P$1 NEWBATT5.P$1
  Bottom 0.508: OLDBATT5.P$1 U$20.P$1
N$96
  pour Top: 245.75,124.71 245.75,138.94 255.4,138.94 255.4,124.71
N$97
  pour Bottom: 245.75,124.71 245.75,138.94 255.4,138.94 255.4,124.71
N$98
  Top 0.508: U$21.P$1 NEWBATT6.P$2
  Bottom 0.508: OLDBATT6.P$2 U$21.P$1
N$99
  Top 0.508: U$22.P$1 NEWBATT6.P$1
  Bottom 0.508: OLDBATT6.P$1 U$22.P$1
N$100
  pour Top: 257.3,124.71 257.3,138.94 266.95,138.94 266.95,124.71
N$101
  pour Bottom: 257.3,124.71 257.3,138.94 266.95,138.94 266.95,124.71
N$169  (via drill 0.38)
  Top 0.254: v62.36,94.89 61.44,93.98 IC12.7
  Bottom 0.254: v62.36,94.89 74.24,94.89 78.56,99.21 90.4,99.21 UNDER_WARN.2
N$170  (via drill 0.38)
  Top 0.254: IC12.5 60.12,91.44 58.9,90.22 58.9,86.31 59.97,85.24 62.81,85.24 68.3,90.73 68.3,107.95 v69.06,108.71
  Bottom 0.254: v69.06,108.71 75.36,108.71 87.3,120.65 UNDER_CRIT.2
N$171  (via drill 0.38)
  Top 0.254: IC12.11 54.94,90.17 54.28,90.83 54.28,92.05 54.94,92.71 IC12.9 56.31,92.76 57.53,92.76 v57.94,93.17
  Bottom 0.254: TEMP_TRIM.2 77.04,93.17 v57.94,93.17
N$172
  Top 0.61: UNDER_CRIT.3 R66.1
N$173
  Top 0.61: UNDER_WARN.3 R67.1
N$174  (via drill 0.38)
  Top 0.254: IC12.4 62.66,90.17 63.32,90.83 63.32,92.05 63.25,92.13 | 63.25,92.13 62.66,92.71 IC12.6 | v67.18,108.71 67.18,99.82 v64.54,97.18 | v63.02,95.66 63.02,95.3 63.32,95 63.32,92.2 63.25,92.13
  Bottom 0.254: v67.18,108.71 UNDER_TRIM.2 | v63.02,95.66 v64.54,97.18
N$175
  Top 0.254: UNDER_TRIM.3 R71.1
N$176
  Top 0.254: TEMP_TRIM.3 R70.1
N$177
  Top 0.254: R72.1 8.15,105.41 5.41,108.15 3.79,108.15 2.31,106.68 UNDERVOLT.A
N$178
  Top 0.254: R73.1 8.15,118.11 5.41,120.85 3.79,120.85 2.31,119.38 UNDERVOLT_WARN.A
N$179
  Top 0.254: R74.1 8.15,92.71 5.41,95.45 3.79,95.45 2.31,93.98 OVERTEMP1.A
N$180
  Top 0.254: R75.1 8.15,86.36 5.41,89.1 3.79,89.1 2.31,87.63 OVERTEMP2.A
N$181
  Top 0.254: R77.1 46.51,114.3 46.51,113.28 41.17,107.95 K3.1
N$182  (via drill 0.38)
  Top 0.254: IC14.9 57.48,110.49 v57.94,110.03 | v71.7,96.27 71.7,90.02 79.12,82.6 CURRENT_TRIM.2
  Bottom 0.254: v71.7,96.27 v57.94,110.03
N$183
  Top 0.61: OVER_WARN.3 R83.1
N$184  (via drill 0.38)
  Top 0.254: IC14.5 62.66,109.22 63.32,109.88 | 63.32,109.88 63.32,111.1 62.66,111.76 IC14.7 | v65.35,107.95 63.42,109.88 63.32,109.88
  Bottom 0.254: v65.35,107.95 OVER_TRIM.2
N$185
  Top 0.254: OVER_TRIM.3 R86.1
N$186
  Top 0.254: CURRENT_TRIM.3 R85.1
N$187
  Top 0.254: R87.1 8.15,99.06 5.41,101.8 3.79,101.8 2.31,100.33 OVERVOLT.A
N$188
  Top 0.254: R88.1 8.15,111.76 5.41,114.5 3.79,114.5 2.31,113.03 OVERVOLT_WARN.A
N$189
  Top 0.254: R89.1 8.15,80.01 5.41,82.75 3.79,82.75 2.31,81.28 OVERCURRENT.A
N$190  (via drill 0.38)
  Top 0.254: OVERCURRENT_FET.4 22.07,82.55 | 22.07,82.55 OVERCURRENT_FET.2 | K3.2 47.32,107.95 v42.8,103.43 | v22.07,82.7 22.07,82.55
  Bottom 0.254: v22.07,82.7 v42.8,103.43
N$191
  Top 0.254: OVERTEMP2_FET.4 20.02,89.03 | 20.02,89.03 23.8,85.24 23.8,84.89 OVERCURRENT_FET.3 | OVERTEMP2_FET.4 | OVERTEMP2_FET.2 22.43,91.44 20.02,89.03
N$192
  Top 0.254: OVERTEMP1_FET.4 20.02,97.92 | 20.02,97.92 23.8,94.13 23.8,93.78 OVERTEMP2_FET.3 | OVERTEMP1_FET.4 | OVERTEMP1_FET.2 22.43,100.33 20.02,97.92
N$193
  Top 0.254: OVERVOLT_FET.4 20.02,106.81 | 20.02,106.81 23.8,103.02 23.8,102.67 OVERTEMP1_FET.3 | OVERVOLT_FET.4 | OVERVOLT_FET.2 22.43,109.22 20.02,106.81
N$194
  Top 0.254: UNDERVOLT_FET.4 20.02,115.7 | 20.02,115.7 23.8,111.91 23.8,111.56 OVERVOLT_FET.3 | UNDERVOLT_FET.4 | UNDERVOLT_FET.2 22.43,118.11 20.02,115.7
N$195  (via drill 0.38)
  Top 0.254: v59.66,110.49 IC14.6 | v80.54,96.37 v73.79,96.37
  Bottom 0.254: v73.79,96.37 v59.66,110.49 | OVER_WARN.2 v80.54,96.37
N$196  (via drill 0.38)
  Top 0.254: v64.29,107.95 IC14.4
  Bottom 0.254: v64.29,107.95 68.2,104.04 90.45,104.04 OVER_CRIT.2
N$197
  Top 0.61: OVER_CRIT.3 R82.1
N$198  (via drill 0.38)
  Top 0.254: v84.61,63.25 84.61,59.69 R84.1 | v53.72,96.32 53.72,110.54 54.94,111.76 IC14.8
  Bottom 0.254: v84.61,63.25 84.61,65.43 v53.72,96.32
N$199  (via drill 0.38)
  Top 0.254: v82.58,69.85 R68.1 | v59.66,92.41 58.7,93.37 58.7,93.47 58.19,93.98 IC12.8
  Bottom 0.254: v82.58,69.85 82.22,69.85 v59.66,92.41
N$200  (via drill 0.38)
  Top 0.254: R69.1 84.15,64.77 v83.29,65.63 | v57.94,90.98 57.48,91.44 IC12.10
  Bottom 0.254: v57.94,90.98 v83.29,65.63
ON
  Top 0.254: IO.1 154.52,134.87 161.76,134.87 163.16,133.48 163.16,132.84 171.03,124.97 R27.2
OVERCURRENT_CRITICAL  (via drill 0.38)
  Top 0.254: IC14.14 54.94,104.14 v54.48,103.68 | v31.01,81.53 30.5,81.03 30.5,80.11 R81.1 24.05,80.01 23.85,80.21 OVERCURRENT_FET.1 23.7,80.31 23.19,80.31 v22.23,81.28
  Bottom 0.254: v54.48,103.68 53.16,103.68 v31.01,81.53 | v22.23,81.28 OVERCURRENT.K
OVERTEMP_CRITICAL1  (via drill 0.38)
  Top 0.254: IC12.14 39.19,86.36 v36.5,89.05 | v33.05,92.61 33.05,94.49 29.84,97.69 R79.1 24.05,97.79 23.85,97.99 OVERTEMP1_FET.1 23.7,97.94 v22.53,96.77
  Bottom 0.254: v36.5,89.05 36.5,89.71 33.6,92.61 v33.05,92.61 | OVERTEMP1.K 19.74,93.98 v22.53,96.77
OVERTEMP_CRITICAL2  (via drill 0.38)
  Top 0.254: IC12.13 52.5,87.63 50.32,89.81 v35.33,89.81 | v31.77,89.81 30.91,88.95 30.56,88.95 R80.1 24.05,88.9 23.85,89.1 OVERTEMP2_FET.1 23.85,89 v22.48,87.63
  Bottom 0.254: v31.77,89.81 v35.33,89.81 | v22.48,87.63 OVERTEMP2.K
OVERVOLT_CRITICAL  (via drill 0.38)
  Top 0.254: v57.94,105.41 IC14.2 | v31.77,106.02 31.17,106.63 30.56,106.63 R78.1 24.05,106.68 23.85,106.88 OVERVOLT_FET.1 23.7,106.83 v22.53,105.66
  Bottom 0.254: v57.94,105.41 54.48,105.41 53.87,106.02 v31.77,106.02 | OVERVOLT.K 17.2,100.33 v22.53,105.66
OVERVOLT_WARNING1  (via drill 0.38)
  Top 0.254: v57.94,104.14 IC14.1
  Bottom 0.254: v57.94,104.14 55.09,104.14 53.98,105.26 31.47,105.26 22.84,113.89 22.84,115.01 22.38,115.47 7.29,115.47 4.85,113.03 OVERVOLT_WARN.K
SIGNALGND  (via drill 0.61)
  Top 0.254: JP8.2 259.59,112.04 259.11,111.56 259.11,108.58 JP14.3 | X3.2 246.96,72.57 245.36,72.57 245.36,86.54 248.49,89.66 R39.2 248.59,89.76 249.5,90.68 262.61,90.68 v262.61,94.34
  Bottom 0.254: JP14.3 262.61,106.83 v262.61,94.34
SIGNALV+
  Top 0.254: R39.1 258.67,89.66 261.31,87.02 261.31,78.92 253.34,78.92 X3.1
  Bottom 0.254: JP7.2 260.86,117.47 JP14.4 260.93,111.02 263.45,108.51 263.45,93.75 259.38,89.69 258.67,89.69 R39.1
SPI_CLK  (via drill 0.38)
  Top 0.254: ADC1.13 110.74,42.19 112.5,43.94 v120.4,43.94 | v123.6,43.31 124.71,42.19 ADC2.13 | ADC3.13 138.68,42.82 v138.2,43.31 | ADC4.13 152.65,42.39 v151.71,43.33
  Bottom 0.254: v120.4,43.94 122.96,43.94 v123.6,43.31 123.7,43.28 124.61,43.28 128.25,46.91 134.09,46.91 137.69,43.31 v138.2,43.31 138.3,43.38 138.89,43.97 151.03,43.97 151.66,43.33 v151.71,43.33 151.82,43.41 154.25,45.85 SV2.10
SPI_CS1  (via drill 0.38)
  Top 0.254: ADC1.10 114.55,40.97 115.37,40.16 116.28,40.16 116.74,40.62 v116.74,41.35
  Bottom 0.254: v116.74,41.35 116.74,41.94 115.77,42.9 115.77,43.51 119.86,47.6 138.86,47.6 139.7,46.76 169.8,46.76 169.98,46.94 173.43,46.94 174.07,46.3 174.07,44.4 SV2.7
SPI_CS2  (via drill 0.38)
  Top 0.254: ADC2.10 128.52,42.19 132.46,46.13 135.51,46.13 137.62,48.23 v157.63,48.23 | SV2.6 v162.97,48.23
  Bottom 0.254: v162.97,48.23 v157.63,48.23
SPI_CS3  (via drill 0.38)
  Top 0.254: ADC3.10 142.49,40.97 143.31,40.16 147.37,40.16 v147.93,40.72
  Bottom 0.254: v147.93,40.72 154.61,40.72 158.19,37.13 170.89,37.13 171.88,38.12 171.88,39.67 SV2.5
SPI_CS4  (via drill 0.38)
  Top 0.254: ADC4.10 156.46,40.97 159.21,38.23 v164.95,38.23
  Bottom 0.254: SV2.4 v164.95,38.23
SPI_DIN  (via drill 0.38)
  Top 0.254: v156.03,43.31 155.19,42.47 ADC4.11 155.14,41.48 155.14,40.92 153.62,39.4 150.88,39.4 v149.88,38.41 | ADC1.11 113.28,40.97 114.76,39.5 117.83,39.5 v119.99,41.66 | v126.14,43.31 127.25,42.19 ADC2.11 127.31,41.48 127.31,40.92 128.98,39.24 139.5,39.24 140.75,40.5 | ADC3.11 141.22,40.97 140.75,40.5 | 140.75,40.5 v142.85,38.41
  Bottom 0.254: v156.03,43.31 157.23,43.31 158.06,44.15 169.6,44.15 SV2.8 | v119.99,41.66 124.48,41.66 v126.14,43.31 | v142.85,38.41 v149.88,38.41
SPI_DOUT  (via drill 0.38)
  Top 0.254: ADC1.12 112.01,42.19 113.03,43.2 v116.51,43.2 | v124.87,44.58 124.87,43.31 125.98,42.19 ADC2.12 126.03,41.48 126.03,40.92 v127.71,39.24 | ADC3.12 139.95,40.97 138.96,39.98 v138.05,39.98 | v148.9,39.14 149.68,39.14 150.6,40.06 153.01,40.06 153.92,40.97 ADC4.12 153.97,41.71 153.97,42.24 154.99,43.26 v154.99,43.31
  Bottom 0.254: v116.51,43.2 118.62,43.2 120.09,44.68 124.77,44.68 v124.87,44.58 | v127.71,39.24 130.73,39.24 131.47,39.98 v138.05,39.98 138.15,39.9 138.91,39.14 v148.9,39.14 | SV2.9 171.98,45.85 170.89,44.76 169.85,44.76 169.8,44.81 156.49,44.81 v154.99,43.31
TEMP1  (via drill 0.38)
  Top 0.254: v74.7,61.87 81.2,68.38 81.2,69.85 R68.2
  Bottom 0.254: v74.7,61.87 65.51,61.87 SV3.1
TEMP2  (via drill 0.38)
  Top 0.254: v78.66,64.77 R69.2
  Bottom 0.254: v78.66,64.77 77.55,64.77 74.65,67.67 68.05,67.67 SV3.4
UNDERVOLT_CRITICAL  (via drill 0.38)
  Top 0.254: 29.69,115.57 24.05,115.57 23.85,115.77 UNDERVOLT_FET.1 23.7,115.72 23.09,115.72 v22.07,114.71 | 29.69,115.57 R76.1 | IC12.2 60.12,87.63 v59.66,88.09 | v49.15,98.6 46.56,98.6 v34.62,110.54 | v31.11,114.05 29.69,115.47 29.69,115.57
  Bottom 0.254: v49.15,98.6 v59.66,88.09 | v31.11,114.05 v34.62,110.54 | UNDERVOLT.K 14.05,106.68 v22.07,114.71
UNDERVOLT_WARNING  (via drill 0.38)
  Top 0.254: IC12.1 60.12,86.36 v59.66,86.82 | v48.9,97.59 44.32,97.59 v35.13,106.78
  Bottom 0.254: v48.9,97.59 v59.66,86.82 | v35.13,106.78 31.73,106.78 19.13,119.38 UNDERVOLT_WARN.K
VREF  (via drill 0.38)
  Top 0.254: 128.5,51.59 128.5,53.34 128.07,53.77 3V.2 | 128.5,51.59 128.5,50.93 6103CAP2.1 | ADC1.15 108.2,42.19 v111.43,45.41 | v127.56,50.75 128.4,51.59 128.5,51.59 | ADC2.15 122.17,40.72 121.64,40.18 121.64,39.57 122.07,39.14 122.71,39.14 v123.44,39.88 | ADC3.15 136.14,42.8 v136.65,43.31 | ADC4.15 150.11,40.62 v149.48,39.98
  Bottom 0.254: 115.11,45.41 116.74,45.41 122.07,50.75 v127.56,50.75 | 115.11,45.41 v111.43,45.41 | 122.77,40.55 122.71,40.62 116.43,40.62 115.11,41.94 115.11,45.41 | 122.77,40.55 v123.44,39.88 | 122.77,40.55 122.86,40.64 129.87,40.64 132.54,43.31 v136.65,43.31 136.75,43.23 140,39.98 v149.48,39.98 149.58,39.9 152.09,39.9 160.27,31.73 SV1.34
VREF1
  Top 0.254: 3V1.2 40.72,122.12 41.12,122.53 6103CAP4.1 44.93,122.48 50.57,122.48 51.79,121.26 58.95,121.26 62.15,118.06 69.72,118.06 R71.2 69.83,118.11 69.83,105.51 R86.2 69.83,105.41 69.83,92.81 R70.2 69.83,92.71 69.83,80.01 R85.2
VREF2
  Top 0.254: JP1.19 JP1.17 JP1.15 JP1.13 JP1.11 77.6,20.7 | 6103CAP6.1 80.39,28.45 77.85,28.45 77.6,28.19 3V2.2 77.6,28.07 77.6,20.7 | 77.6,20.7 77.6,19.94 JP1.9 JP1.7 JP1.5 JP1.3 JP1.1
VREF3
  Top 0.254: JP1.39 JP1.37 JP1.35 JP1.33 JP1.31 JP1.29 53.34,19.3 53.34,21.34 | 6103CAP8.1 56.26,28.45 53.72,28.45 53.47,28.19 3V3.2 53.34,28.07 53.34,21.34 | 53.34,21.34 JP1.27 JP1.25 JP1.23 JP1.21
VREF4
  Top 0.254: JP1.59 JP1.57 JP1.55 JP1.53 JP1.51 JP1.49 27.94,19.3 27.94,21.34 | 6103CAP10.1 30.86,28.45 28.32,28.45 28.07,28.19 3V4.2 27.94,28.07 27.94,21.34 | 27.94,21.34 JP1.47 JP1.45 JP1.43 JP1.41

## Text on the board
Top: Solar Jackets BareBones BMS | 11/12/2012 REV 1 | 10/12/12 | AIR GAP BOARD REV 2 | SOLAR JACKETS | SOLAR JACKETS ADC BOARD | 11/10/2012 REV 2 | Solar Jackets Blinker Board / Rev 2 11/13/12 | Solar Jackets Power Distribution Board / 10/13/12 REV 2
tNames: DangerousPrototypes.com | FT2232H Breakout Board v1a | JER | IAN | CC-0 | 2010 | VREF | 2 | AGND | 31 | DGND
bNames: EEDATA | FT2232H Breakout Board v1a | Dangerous Prototypes | dangerousprototypes.com | Fulfillment By: | Seeed Studio | seeedstudio.com | !RESET | EECLK | ACBUS7 | EECS | ACBUS6 | BDBUS0 | ACBUS5 | BDBUS1 | ACBUS4 | BDBUS2 | ACBUS3 | BDBUS3 | ACBUS2 | BDBUS4 | ACBUS1 | BDBUS5 | ACBUS0 | BDBUS6 | ADBUS7 | BDBUS7 | ADBUS6 | BCBUS0 | ADBUS5 | BCBUS1 | ADBUS4 | BCBUS2 | ADBUS3 | BCBUS3 | ADBUS2 | BCBUS4 | ADBUS1 | BCBUS5 | ADBUS0 | BCBUS6 | !RESET | BCBUS7 | GND | !PWEREN | 1.8V | GND | 3.3V | 3V3 | 5V
tValues: - | + | ON | DIR | 6A4 | 6A4 | + | - | In | 96V | 12V | 5V | TEMP2 | Gnd | 5V | Gnd | Gnd | Out | 5V | Gnd | Gnd | CURR | TEMP1 | DOUT | CLK | DIN | CS1 | 2 | 3 | GND | 4 | GND | 12V | VREF1 | VREF2 | VREF3 | 12V / / LED + / / LED + / / LED + / / LED + / / LED + / / LED + / / LED + / / BLNK_R IN / / REGEN IN | <-GND-> | GND / / BLNK_R / / BLNK_R / / BLNK_L / / BLNK_L / / BRAKE / / BRAKE / / BRAKE / / BLNK_L IN / / BRAKE IN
